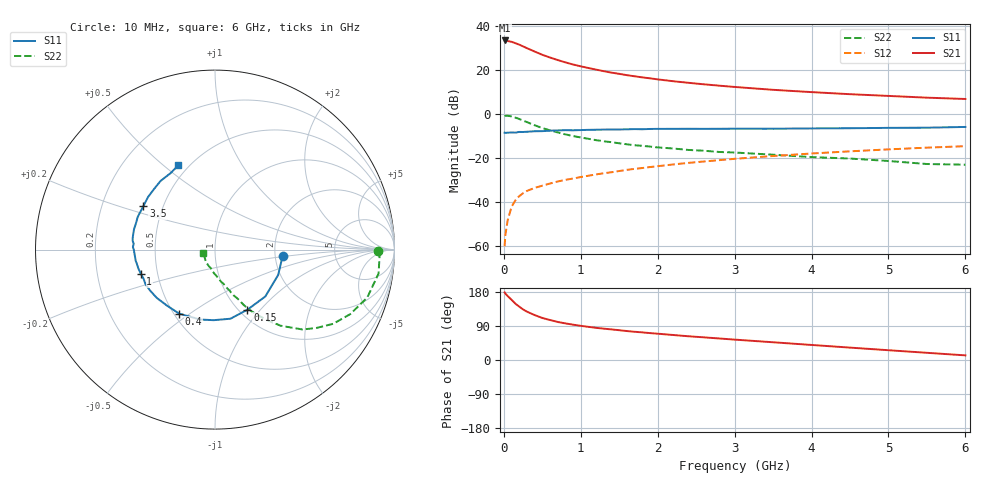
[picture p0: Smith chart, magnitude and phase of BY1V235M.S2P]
! SIEMENS Small Signal Semiconductors
! BFY420
! Si NPN RF SIEGET Grounded Emitter Transistor in MICRO-X
! VCE = 1.25 V  IC = 35 mA
! Common Emitter S-Parameters:  October  1996
# GHz  S  MA  R  50
!  f  S11  S21  S12  S22
! GHz  MAG  ANG  MAG  ANG  MAG  ANG  MAG  ANG
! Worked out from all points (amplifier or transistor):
!   36 points, 10 MHz to 6 GHz, reference 50 ohm
!   highest |S21| = 33.5 dB at 10 MHz (marker M1)
!   |S21| within 3 dB of that: start of sweep to 268.5 MHz
!   unconditionally stable (mu >= 1): start of sweep to 15.81 MHz; 1.328 GHz to end of sweep
!   at 250 MHz: K = 0.42, MSG = 33.4 dB, |S12| = -35.9 dB
!   at 1.4 GHz: K = 1.02, MAG = 21.8 dB, |S12| = -26.4 dB
!   at 6 GHz: K = 1.09, MAG = 8.9 dB, |S12| = -14.6 dB
!   S11 on the Smith chart (normalised r, x): 10 MHz: 2.20, -0.19; 150 MHz: 1.09, -0.85; 400 MHz: 0.53, -0.46; 1 GHz: 0.40, -0.13; 3.5 GHz: 0.39, +0.24; 6 GHz: 0.44, +0.56
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0.01  0.3793 -5.7  47.32 178.4  0.001 113.7  0.9106 -0.5
0.02  0.3754 -10.2  47.19 175.0  0.0018 84.2  0.9173 -2.4
0.05  0.3793 -21.8  45.88 168.8  0.0039 80.5  0.9212 -8.3
0.1  0.3831 -43.0  44.16 158.8  0.0078 79.3  0.8893 -17.5
0.15  0.3804 -61.6  41.06 148.6  0.011 70.1  0.8349 -25.5
0.2  0.3946 -77.4  38.05 140.9  0.0137 67.9  0.7778 -32.1
0.25  0.3933 -91.1  34.65 133.4  0.016 63.7  0.7128 -37.8
0.3  0.3983 -102.0  31.63 127.6  0.018 62.7  0.6601 -42.4
0.4  0.4089 -119.2  26.5 118.6  0.0211 59.3  0.5604 -49.2
0.5  0.4112 -131.0  22.36 110.9  0.0237 58.9  0.4846 -53.8
0.6  0.4215 -140.3  19.36 105.5  0.0265 59.3  0.4282 -57.4
0.7  0.4274 -147.6  16.99 100.4  0.0295 60.1  0.3846 -60.4
0.8  0.4326 -153.4  15.03 96.6  0.0322 58.7  0.3471 -62.6
1  0.435 -162.0  12.21 90.2  0.0373 60.5  0.2954 -65.7
1.1  0.4401 -166.5  11.18 87.5  0.0399 60.3  0.2752 -67.9
1.3  0.4463 -171.9  9.475 82.7  0.0455 60.1  0.2419 -70.4
1.6  0.4523 -179.8  7.693 76.4  0.0543 60.2  0.2066 -74.9
2.2  0.4639 168.8  5.61 66.0  0.072 57.5  0.166 -82.5
3.5  0.4667 148.8  3.574 46.8  0.112 48.8  0.1199 -97.6
4.5  0.4788 135.2  2.843 32.7  0.1429 39.4  0.098 -110.6
5.5  0.4927 120.1  2.371 19.0  0.1734 29.5  0.0736 -140.6
6  0.5125 113.4  2.212 12.2  0.1872 24.3  0.0711 -162.7
